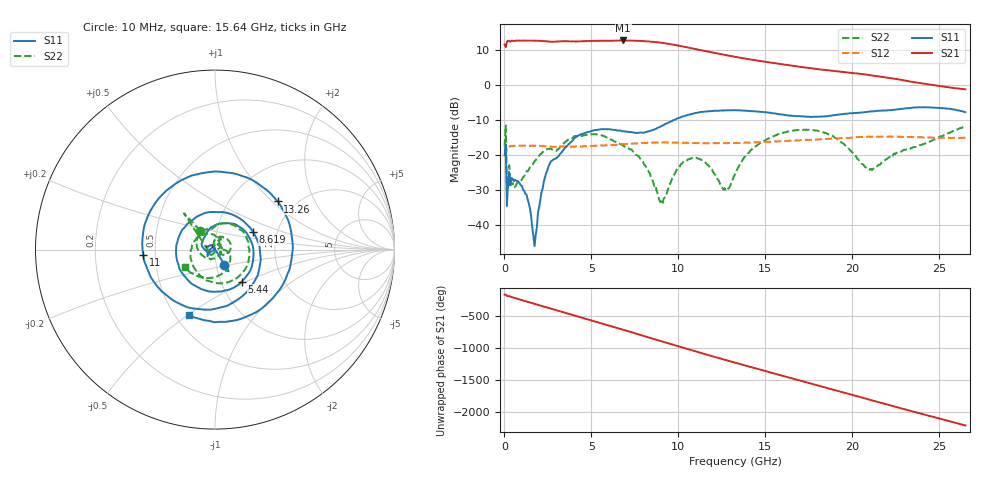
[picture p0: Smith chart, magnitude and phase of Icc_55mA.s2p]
!Keysight Technologies,N5245A,MY52451697,A.10.60.06
!Date: Thursday, May 06, 2021 15:04:33
!Correction: S11(Full 2 Port(1,4))
!S41(Full 2 Port(1,4))
!S14(Full 2 Port(1,4))
!S44(Full 2 Port(1,4))
!S2P File: Measurements: S11, S41, S14, S44:
# Hz S  dB  R 50
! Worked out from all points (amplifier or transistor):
!   401 points, 10 MHz to 26.5 GHz, reference 50 ohm
!   highest |S21| = 12.8 dB at 6.831 GHz (marker M1)
!   |S21| within 3 dB of that: start of sweep to 11.5 GHz
!   unconditionally stable (mu >= 1): start of sweep to end of sweep
!   at 4.381 GHz: K = 1.13, MAG = 12.8 dB, |S12| = -17.5 dB
!   at 13.26 GHz: K = 1.23, MAG = 9.4 dB, |S12| = -16.5 dB
!   at 26.5 GHz: K = 2.49, MAG = 0.1 dB, |S12| = -15.0 dB
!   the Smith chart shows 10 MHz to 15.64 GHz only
!   S11 on the Smith chart (normalised r, x): 10 MHz: 1.09, -0.19; 5.44 GHz: 1.25, -0.47; 8.619 GHz: 1.50, +0.31; 11 GHz: 0.43, -0.03; 13.26 GHz: 1.63, +1.08; 15.64 GHz: 0.59, -0.51
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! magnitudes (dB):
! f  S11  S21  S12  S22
! 10 MHz  -20.1  11.6  -18.3  -17.5
! 274.9 MHz  -25.0  12.6  -17.4  -22.8
! 473.6 MHz  -26.7  12.7  -17.4  -28.0
! 1.268 GHz  -31.3  12.7  -17.3  -24.6
! 1.732 GHz  -46.0  12.7  -17.3  -21.7
! 2.593 GHz  -22.5  12.5  -17.6  -18.2
! 4.447 GHz  -14.0  12.6  -17.6  -14.6
! 5.44 GHz  -12.7  12.7  -17.3  -14.1
! 6.831 GHz  -13.1  12.8  -16.8  -17.3
! 8.619 GHz  -12.6  12.4  -16.4  -28.8
! 8.884 GHz  -12.0  12.2  -16.3  -32.5
! 9.149 GHz  -11.4  12.1  -16.3  -32.5
! 10.21 GHz  -9.0  11.1  -16.5  -22.3
! 11 GHz  -7.9  10.3  -16.5  -20.7
! 12.66 GHz  -7.2  8.7  -16.5  -29.4
! 13.26 GHz  -7.1  8.1  -16.5  -25.5
! 14.25 GHz  -7.4  7.3  -16.3  -18.2
! 15.64 GHz  -8.1  6.2  -16.1  -14.2
! 17.69 GHz  -9.0  4.8  -15.6  -12.8
! 20.87 GHz  -7.6  3.0  -14.7  -23.7
! 22.13 GHz  -7.1  2.1  -14.6  -20.5
! 26.5 GHz  -7.7  -1.2  -15.0  -11.8
